| TEXAS INSTRUMENTS INCORPORATED
| Standard Linear and Logic Group
| IBIS Model of SN74ABT162244
| 16-BIT BUFFER/DRIVER WITH 3-STATE OUTPUTS
| This file contains package information for the following:
|  SSOP 48-pin (DL) package as [Component] ABT162244G_DL
|  TSSOP 48-pin (DGG) package as [Component] ABT162244G_DGG
|  TVSOP 48-pin (DGV) package as [Component] ABT162244G_DGV
| This device can be powered at the following Vccs:
|  5 volt Vcc
| This file provides unique models under the [Model Selector] for each Vcc.
| For operation at a specific Vcc, select the appropriate model after each
| [Model Selector] keyword.
[IBIS Ver]   3.2
[Comment char]  |_char
[File Name]   sn74abt162244.ibs
[File Rev]   1.1 | g_die
[Date]   May 28, 2009
[Source]   Data created from TI-SPICE simulations at TI-SLL.
[Notes]   The following is an IBIS list for the SN74ABT162244.
   Please contact sllibis@ti.com with questions and
   comments concerning SLL IBIS models.
   - FILE REV HISTORY
   - 1.1 Release IBIS file on 05/28/09
   - Power clamp data deleted from control input model as there
   is no power-clamp diode.
[Disclaimer] Property of Texas Instruments Incorporated.  Unauthorized
   reproduction and/or distribution is strictly prohibited.
   This product is protected under copyright law.
   Created  2009, (C) Copyright  2009, Texas Instruments
   Incorporated, All Rights Reserved
   UNLESS THERE IS A SIGNED, WRITTEN AGREEMENT TO THE
   CONTRARY, TEXAS INSTRUMENTS (TI) IS PROVIDING THE IBIS
   MODELS  AND WITHOUT ANY WARRANTY, EXPRESSED OR
   IMPLIED.  TI assumes no liability for:
   1) the accuracy of the IBIS models provided to your
   company;
   2) the proper functioning of these IBIS Models in your
   design or for any resulting applications; or
   3) infringement of patents, copyrights or intellectual
   property rights resulting from your use of these IBIS
   models.
   TI provides IBIS Models as a service to our customers.
   You and your company shall not distribute, sell or give
   these models to anyone else without prior written
   permission from TI.
   TI reserves the right to make changes to our products or
   to discontinue any semiconductor product or service
   without notice, and advises our customers to obtain the
   latest version of relevant information to verify, before
   placing orders, that the information being relied on is
   current.
   Please be aware that your receipt and use of the IBIS
   information provided shall serve as acceptance of these
   terms and conditions.  If you do not accept these terms,
   you should return or destroy the IBIS models and any
   other accompanying information immediately.
| Component SN74ABT162244_DL 48-PIN SSOP
[Component]   SN74ABT162244_DL
[Manufacturer]   Texas Instruments, Inc.
[Package]
|   typ   min   max
R_pkg   4.800e-02   3.800e-02   5.300e-02
L_pkg   6.046e-09   5.084e-09   7.968e-09
C_pkg   8.130e-13   5.690e-13   1.157e-12
[Pin]   signal_name   model_name   R_pin   L_pin   C_pin
1   1OE   ABT162244G_OE_IN_50  4.600e-02   7.968e-09   1.017e-12
2   1Y1   ABT162244G_OUT_50   4.400e-02   7.299e-09   1.157e-12
3   1Y2   ABT162244G_OUT_50   4.300e-02   6.765e-09   1.058e-12
4   GND   GND   4.100e-02   6.269e-09   9.330e-13
5   1Y3   ABT162244G_OUT_50   3.800e-02   5.856e-09   8.290e-13
6   1Y4   ABT162244G_OUT_50   4.600e-02   5.802e-09   7.900e-13
7   VCC   POWER   5.000e-02   5.656e-09   7.380e-13
8   2Y1   ABT162244G_OUT_50   5.300e-02   5.500e-09   6.430e-13
9   2Y2   ABT162244G_OUT_50   5.200e-02   5.304e-09   6.060e-13
10   GND   GND   5.300e-02   5.189e-09   5.830e-13
11   2Y3   ABT162244G_OUT_50   5.100e-02   5.084e-09   5.690e-13
12   2Y4   ABT162244G_OUT_50   5.300e-02   5.862e-09   8.330e-13
13   3Y1   ABT162244G_OUT_50   5.300e-02   5.862e-09   8.330e-13
14   3Y2   ABT162244G_OUT_50   5.100e-02   5.084e-09   5.690e-13
15   GND   GND   5.300e-02   5.189e-09   5.830e-13
16   3Y3   ABT162244G_OUT_50   5.200e-02   5.304e-09   6.060e-13
17   3Y4   ABT162244G_OUT_50   5.300e-02   5.500e-09   6.430e-13
18   VCC   POWER   5.000e-02   5.656e-09   7.380e-13
19   4Y1   ABT162244G_OUT_50   4.600e-02   5.802e-09   7.900e-13
20   4Y2   ABT162244G_OUT_50   3.800e-02   5.856e-09   8.290e-13
21   GND   GND   4.100e-02   6.269e-09   9.330e-13
22   4Y3   ABT162244G_OUT_50   4.300e-02   6.765e-09   1.058e-12
23   4Y4   ABT162244G_OUT_50   4.400e-02   7.299e-09   1.157e-12
24   4OE   ABT162244G_IN_50   4.600e-02   7.968e-09   1.017e-12
25   3OE   ABT162244G_IN_50   4.600e-02   7.968e-09   1.017e-12
26   4A4   ABT162244G_IN_50   4.400e-02   7.299e-09   1.157e-12
27   4A3   ABT162244G_IN_50   4.300e-02   6.765e-09   1.058e-12
28   GND   GND   4.100e-02   6.269e-09   9.330e-13
29   4A2   ABT162244G_IN_50   3.800e-02   5.856e-09   8.290e-13
30   4A1   ABT162244G_IN_50   4.600e-02   5.802e-09   7.900e-13
31   VCC   POWER   5.000e-02   5.656e-09   7.380e-13
32   3A4   ABT162244G_IN_50   5.300e-02   5.500e-09   6.430e-13
33   3A3   ABT162244G_IN_50   5.200e-02   5.304e-09   6.060e-13
34   GND   GND   5.300e-02   5.189e-09   5.830e-13
35   3A2   ABT162244G_IN_50   5.100e-02   5.084e-09   5.690e-13
36   3A1   ABT162244G_IN_50   5.300e-02   5.862e-09   8.330e-13
37   2A4   ABT162244G_IN_50   5.300e-02   5.862e-09   8.330e-13
38   2A3   ABT162244G_IN_50   5.100e-02   5.084e-09   5.690e-13
39   GND   GND   5.300e-02   5.189e-09   5.830e-13
40   2A2   ABT162244G_IN_50   5.200e-02   5.304e-09   6.060e-13
41   2A1   ABT162244G_IN_50   5.300e-02   5.500e-09   6.430e-13
42   VCC   POWER   5.000e-02   5.656e-09   7.380e-13
43   1A4   ABT162244G_IN_50   4.600e-02   5.802e-09   7.900e-13
44   1A3   ABT162244G_IN_50   3.800e-02   5.856e-09   8.290e-13
45   GND   GND   4.100e-02   6.269e-09   9.330e-13
46   1A2   ABT162244G_IN_50   4.300e-02   6.765e-09   1.058e-12
47   1A1   ABT162244G_IN_50   4.400e-02   7.299e-09   1.157e-12
48   2OE   ABT162244G_OE_IN_50  4.600e-02   7.967e-09   1.017e-12
| Component SN74ABT162244_DGG 48-PIN TSSOP
[Component]   SN74ABT162244_DGG
[Manufacturer]   Texas Instruments, Inc.
[Package]
|   typ   min   max
R_pkg   6.200e-02   5.000e-02   7.800e-02
L_pkg   3.527e-09   3.128e-09   4.255e-09
C_pkg   5.300e-13   4.170e-13   6.850e-13
[Pin]   signal_name   model_name   R_pin   L_pin   C_pin
1   1OE   ABT162244G_OE_IN_50  5.000e-02   4.250e-09   6.710e-13
2   1Y1   ABT162244G_OUT_50   5.700e-02   3.956e-09   6.740e-13
3   1Y2   ABT162244G_OUT_50   7.100e-02   3.922e-09   6.190e-13
4   GND   GND   7.800e-02   3.841e-09   6.180e-13
5   1Y3   ABT162244G_OUT_50   5.600e-02   3.535e-09   5.550e-13
6   1Y4   ABT162244G_OUT_50   5.800e-02   3.464e-09   5.030e-13
7   VCC   POWER   6.000e-02   3.362e-09   4.980e-13
8   2Y1   ABT162244G_OUT_50   6.100e-02   3.293e-09   4.620e-13
9   2Y2   ABT162244G_OUT_50   6.300e-02   3.240e-09   4.550e-13
10   GND   GND   6.300e-02   3.175e-09   4.420e-13
11   2Y3   ABT162244G_OUT_50   6.400e-02   3.153e-09   4.290e-13
12   2Y4   ABT162244G_OUT_50   6.500e-02   3.128e-09   4.180e-13
13   3Y1   ABT162244G_OUT_50   6.500e-02   3.128e-09   4.180e-13
14   3Y2   ABT162244G_OUT_50   6.400e-02   3.154e-09   4.290e-13
15   GND   GND   6.300e-02   3.174e-09   4.420e-13
16   3Y3   ABT162244G_OUT_50   6.300e-02   3.241e-09   4.550e-13
17   3Y4   ABT162244G_OUT_50   6.100e-02   3.293e-09   4.620e-13
18   VCC   POWER   6.000e-02   3.362e-09   4.970e-13
19   4Y1   ABT162244G_OUT_50   5.800e-02   3.464e-09   5.030e-13
20   4Y2   ABT162244G_OUT_50   5.600e-02   3.537e-09   5.600e-13
21   GND   GND   7.700e-02   3.839e-09   6.260e-13
22   4Y3   ABT162244G_OUT_50   7.100e-02   3.917e-09   6.270e-13
23   4Y4   ABT162244G_OUT_50   5.800e-02   3.955e-09   6.850e-13
24   4OE   ABT162244G_IN_50   5.200e-02   4.255e-09   6.790e-13
25   3OE   ABT162244G_IN_50   5.100e-02   4.254e-09   6.760e-13
26   4A4   ABT162244G_IN_50   5.800e-02   3.957e-09   6.790e-13
27   4A3   ABT162244G_IN_50   7.100e-02   3.920e-09   6.210e-13
28   GND   GND   7.800e-02   3.843e-09   6.220e-13
29   4A2   ABT162244G_IN_50   5.600e-02   3.539e-09   5.600e-13
30   4A1   ABT162244G_IN_50   5.800e-02   3.466e-09   5.030e-13
31   VCC   POWER   6.000e-02   3.363e-09   4.970e-13
32   3A4   ABT162244G_IN_50   6.100e-02   3.294e-09   4.620e-13
33   3A3   ABT162244G_IN_50   6.300e-02   3.241e-09   4.540e-13
34   GND   GND   6.300e-02   3.175e-09   4.410e-13
35   3A2   ABT162244G_IN_50   6.400e-02   3.153e-09   4.290e-13
36   3A1   ABT162244G_IN_50   6.500e-02   3.129e-09   4.170e-13
37   2A4   ABT162244G_IN_50   6.500e-02   3.129e-09   4.170e-13
38   2A3   ABT162244G_IN_50   6.400e-02   3.152e-09   4.290e-13
39   GND   GND   6.400e-02   3.176e-09   4.410e-13
40   2A2   ABT162244G_IN_50   6.300e-02   3.241e-09   4.540e-13
41   2A1   ABT162244G_IN_50   6.100e-02   3.293e-09   4.620e-13
42   VCC   POWER   6.000e-02   3.363e-09   4.970e-13
43   1A4   ABT162244G_IN_50   5.800e-02   3.464e-09   5.030e-13
44   1A3   ABT162244G_IN_50   5.600e-02   3.534e-09   5.610e-13
45   GND   GND   7.800e-02   3.841e-09   6.260e-13
46   1A2   ABT162244G_IN_50   7.100e-02   3.920e-09   6.220e-13
47   1A1   ABT162244G_IN_50   5.700e-02   3.955e-09   6.770e-13
48   2OE   ABT162244G_OE_IN_50  5.100e-02   4.252e-09   6.720e-13
| Component SN74ABT162244_DGV 48-PIN TVSOP
[Component]   SN74ABT162244_DGV
[Manufacturer]   Texas Instruments, Inc.
[Package]
|   typ   min   max
R_pkg   1.370e-01   1.010e-01   1.720e-01
L_pkg   3.632e-09   2.739e-09   5.243e-09
C_pkg   5.430e-13   4.100e-13   7.930e-13
[Pin]   signal_name   model_name   R_pin   L_pin   C_pin
1   1OE   ABT162244G_OE_IN_50  1.680e-01   5.238e-09   7.750e-13
2   1Y1   ABT162244G_OUT_50   1.660e-01   4.546e-09   6.740e-13
3   1Y2   ABT162244G_OUT_50   1.700e-01   4.356e-09   6.200e-13
4   GND   GND   1.720e-01   4.192e-09   5.310e-13
5   1Y3   ABT162244G_OUT_50   1.570e-01   3.821e-09   5.020e-13
6   1Y4   ABT162244G_OUT_50   1.430e-01   3.623e-09   5.600e-13
7   VCC   POWER   1.300e-01   3.292e-09   5.060e-13
8   2Y1   ABT162244G_OUT_50   1.190e-01   3.090e-09   4.520e-13
9   2Y2   ABT162244G_OUT_50   1.110e-01   2.927e-09   4.440e-13
10   GND   GND   1.050e-01   2.807e-09   4.350e-13
11   2Y3   ABT162244G_OUT_50   1.010e-01   2.739e-09   4.260e-13
12   2Y4   ABT162244G_OUT_50   1.020e-01   2.949e-09   5.040e-13
13   3Y1   ABT162244G_OUT_50   1.020e-01   2.960e-09   4.800e-13
14   3Y2   ABT162244G_OUT_50   1.010e-01   2.747e-09   4.100e-13
15   GND   GND   1.050e-01   2.809e-09   4.350e-13
16   3Y3   ABT162244G_OUT_50   1.110e-01   2.928e-09   4.440e-13
17   3Y4   ABT162244G_OUT_50   1.190e-01   3.090e-09   4.520e-13
18   VCC   POWER   1.300e-01   3.293e-09   5.120e-13
19   4Y1   ABT162244G_OUT_50   1.430e-01   3.622e-09   5.750e-13
20   4Y2   ABT162244G_OUT_50   1.570e-01   3.818e-09   5.200e-13
21   GND   GND   1.720e-01   4.186e-09   5.560e-13
22   4Y3   ABT162244G_OUT_50   1.700e-01   4.354e-09   6.430e-13
23   4Y4   ABT162244G_OUT_50   1.660e-01   4.544e-09   6.970e-13
24   4OE   ABT162244G_IN_50   1.680e-01   5.240e-09   7.930e-13
25   3OE   ABT162244G_IN_50   1.680e-01   5.243e-09   7.900e-13
26   4A4   ABT162244G_IN_50   1.660e-01   4.544e-09   6.940e-13
27   4A3   ABT162244G_IN_50   1.700e-01   4.351e-09   6.460e-13
28   GND   GND   1.720e-01   4.185e-09   5.630e-13
29   4A2   ABT162244G_IN_50   1.570e-01   3.817e-09   5.270e-13
30   4A1   ABT162244G_IN_50   1.430e-01   3.622e-09   5.790e-13
31   VCC   POWER   1.300e-01   3.293e-09   5.140e-13
32   3A4   ABT162244G_IN_50   1.190e-01   3.091e-09   4.560e-13
33   3A3   ABT162244G_IN_50   1.110e-01   2.928e-09   4.480e-13
34   GND   GND   1.050e-01   2.810e-09   4.380e-13
35   3A2   ABT162244G_IN_50   1.010e-01   2.748e-09   4.140e-13
36   3A1   ABT162244G_IN_50   1.020e-01   2.959e-09   4.830e-13
37   2A4   ABT162244G_IN_50   1.020e-01   2.949e-09   5.080e-13
38   2A3   ABT162244G_IN_50   1.010e-01   2.739e-09   4.300e-13
39   GND   GND   1.050e-01   2.806e-09   4.380e-13
40   2A2   ABT162244G_IN_50   1.110e-01   2.927e-09   4.480e-13
41   2A1   ABT162244G_IN_50   1.190e-01   3.091e-09   4.560e-13
42   VCC   POWER   1.300e-01   3.292e-09   5.110e-13
43   1A4   ABT162244G_IN_50   1.430e-01   3.623e-09   5.700e-13
44   1A3   ABT162244G_IN_50   1.570e-01   3.820e-09   5.150e-13
45   GND   GND   1.720e-01   4.189e-09   5.500e-13
46   1A2   ABT162244G_IN_50   1.700e-01   4.356e-09   6.370e-13
47   1A1   ABT162244G_IN_50   1.660e-01   4.547e-09   6.930e-13
48   2OE   ABT162244G_OE_IN_50  1.680e-01   5.233e-09   7.900e-13
| Models and submodels in the file (3): ABT162244G_IN_50 (Input), ABT162244G_OE_IN_50 (Input), ABT162244G_OUT_50 (3-state)
